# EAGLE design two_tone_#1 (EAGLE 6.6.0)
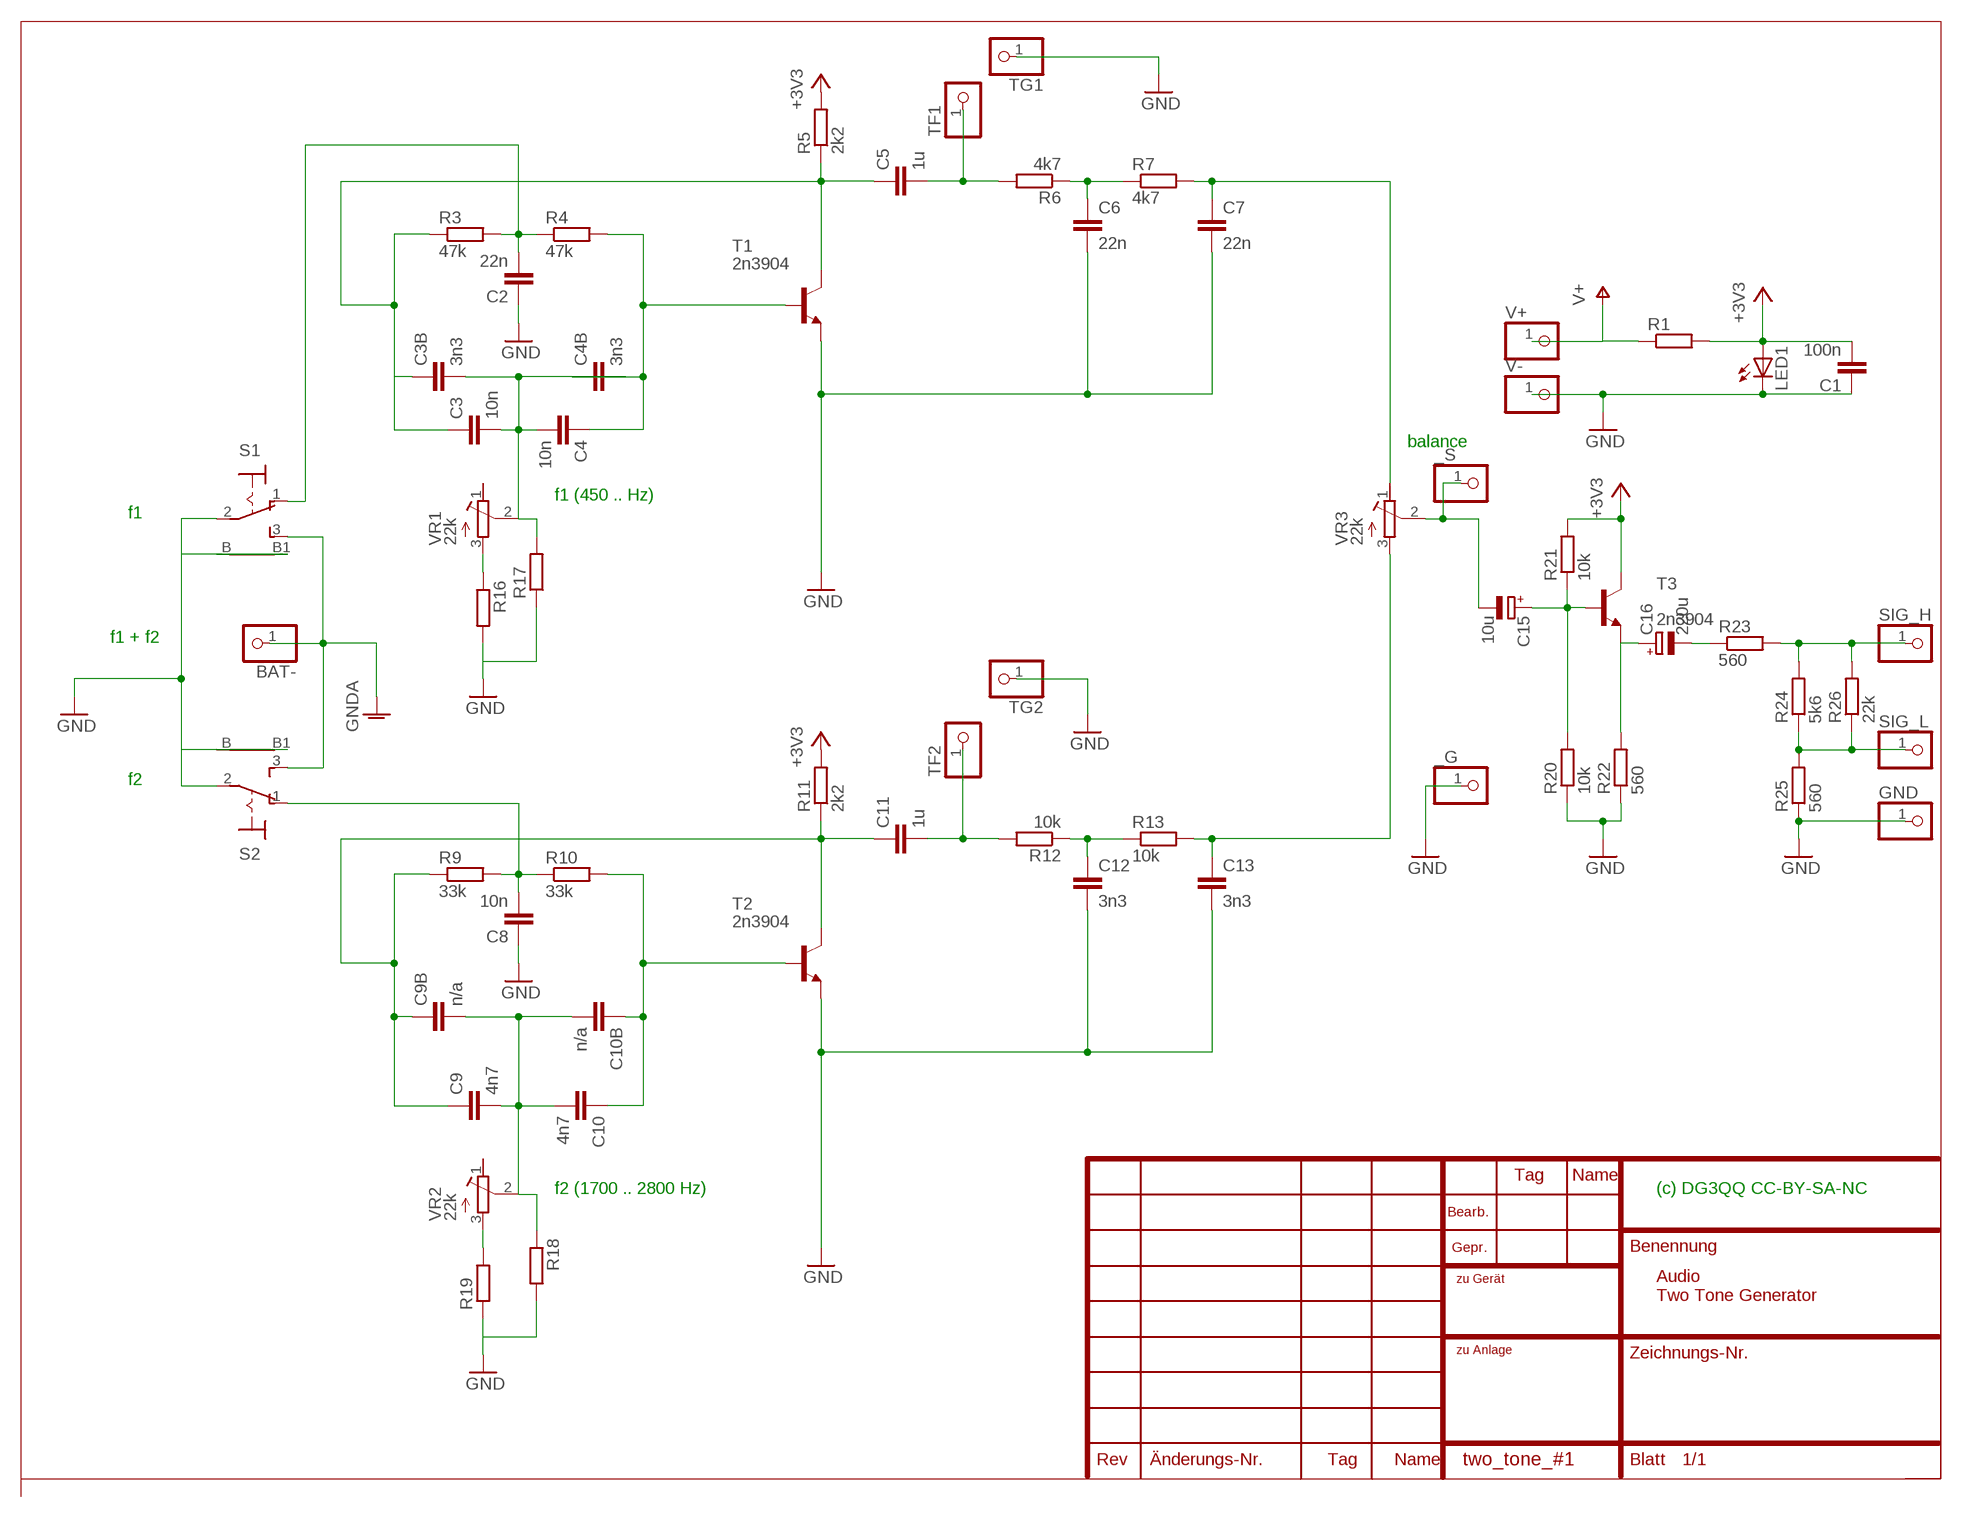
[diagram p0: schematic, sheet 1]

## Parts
_G  PINHD-1X1  [1X01]
_S  PINHD-1X1  [1X01]
BAT-  PINHD-1X1  [1X01]
C1  100n  C-EU025_050-025X075  [C025_050-025X075]
C2  22n  C-EU025_050-025X075  [C025_050-025X075]
C3  10n  C-EU025_050-025X075  [C025_050-025X075]
C3B  3n3  C-EU025_050-025X075  [C025_050-025X075]
C4  10n  C-EU025_050-025X075  [C025_050-025X075]
C4B  3n3  C-EU025_050-025X075  [C025_050-025X075]
C5  1u  C-EU025_050-025X075  [C025_050-025X075]
C6  22n  C-EU025_050-025X075  [C025_050-025X075]
C7  22n  C-EU025_050-025X075  [C025_050-025X075]
C8  10n  C-EU025_050-025X075  [C025_050-025X075]
C9  4n7  C-EU025_050-025X075  [C025_050-025X075]
C9B  n/a  C-EU025_050-025X075  [C025_050-025X075]
C10  4n7  C-EU025_050-025X075  [C025_050-025X075]
C10B  n/a  C-EU025_050-025X075  [C025_050-025X075]
C11  1u  C-EU025_050-025X075  [C025_050-025X075]
C12  3n3  C-EU025_050-025X075  [C025_050-025X075]
C13  3n3  C-EU025_050-025X075  [C025_050-025X075]
C15  10u  CPOL-EUE2.5-5  [E2,5-5]
C16  220u  CPOL-EUE5-10.5  [E5-10,5]
GND  PINHD-1X1  [1X01]
LED1  LED3MM  [LED3MM]
R1  R-EU_0207/2V  [0207/2V]
R3  47k  R-EU_0207/10  [0207/10]
R4  47k  R-EU_0207/2V  [0207/2V]
R5  2k2  R-EU_0207/2V  [0207/2V]
R6  4k7  R-EU_0207/2V  [0207/2V]
R7  4k7  R-EU_0207/2V  [0207/2V]
R9  33k  R-EU_0207/10  [0207/10]
R10  33k  R-EU_0207/2V  [0207/2V]
R11  2k2  R-EU_0207/2V  [0207/2V]
R12  10k  R-EU_0207/2V  [0207/2V]
R13  10k  R-EU_0207/2V  [0207/2V]
R16  R-EU_0207/2V  [0207/2V]
R17  R-EU_0207/2V  [0207/2V]
R18  R-EU_0207/2V  [0207/2V]
R19  R-EU_0207/2V  [0207/2V]
R20  10k  R-EU_0207/2V  [0207/2V]
R21  10k  R-EU_0207/2V  [0207/2V]
R22  560  R-EU_0207/2V  [0207/2V]
R23  560  R-EU_0207/2V  [0207/2V]
R24  5k6  R-EU_0207/2V  [0207/2V]
R25  560  R-EU_0207/2V  [0207/2V]
R26  22k  R-EU_0207/2V  [0207/2V]
S1  9070-1W  [9070-1W]
S2  9070-1W  [9070-1W]
SIG_H  PINHD-1X1  [1X01]
SIG_L  PINHD-1X1  [1X01]
T1  2n3904  2N3904-NPN-TO92-EBC  [TO92-EBC]
T2  2n3904  2N3904-NPN-TO92-EBC  [TO92-EBC]
T3  2n3904  2N3904-NPN-TO92-EBC  [TO92-EBC]
TF1  PINHD-1X1  [1X01]
TF2  PINHD-1X1  [1X01]
TG1  PINHD-1X1  [1X01]
TG2  PINHD-1X1  [1X01]
V+  PINHD-1X1  [1X01]
V-  PINHD-1X1  [1X01]
VR1  22k  R-TRIMM_414S6  [SPINDLE_414S6]
VR2  22k  R-TRIMM_414S6  [SPINDLE_414S6]
VR3  22k  R-TRIMM_414S6  [SPINDLE_414S6]

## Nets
+3V3: C1.2 LED1.A R1.2 R5.2 R11.2 R21.2 T3.C
BAT-: BAT-.1 S1.3(S) S2.3(S) ; supply symbol labelled GNDA
GND: _G.1 C1.1 C2.1 C6.2 C7.2 C8.1 C12.2 C13.2 GND.1 LED1.K(C) R16.2 R17.1 R18.2 R19.1 R20.1 R22.1 R25.1 S1.2(P) S1.B S1.B1 S2.2(P) S2.B S2.B1 T1.E T2.E TG1.1 TG2.1 V-.1
N$1: C5.2 R6.2 TF1.1
N$2: C6.1 R6.1 R7.1
N$3: C2.2 R3.2 R4.1 S1.1(O)
N$4: C4.1 C4B.1 R4.2 T1.B
N$5: C3.1 C3B.1 C5.1 R3.1 R5.1 T1.C
N$6: C3.2 C3B.2 C4.2 C4B.2 R17.2 VR1.2(S)
N$7: C7.1 R7.2 VR3.1(A)
N$8: C8.2 R9.2 R10.1 S2.1(O)
N$9: C10.1 C10B.1 R10.2 T2.B
N$10: C9.1 C9B.1 C11.1 R9.1 R11.1 T2.C
N$11: C9.2 C9B.2 C10.2 C10B.2 R18.1 VR2.2(S)
N$12: C11.2 R12.2 TF2.1
N$13: C12.1 R12.1 R13.1
N$14: C13.1 R13.2 VR3.3(E)
N$15: R19.2 VR2.3(E)
N$16: C15.+ R20.2 R21.1 T3.B
N$17: _S.1 C15.- VR3.2(S)
N$19: R16.1 VR1.3(E)
N$20: C16.+ R22.2 T3.E
N$23: C16.- R23.1
N$24: R23.2 R24.2 R26.2 SIG_H.1
N$25: R24.1 R25.2 R26.1 SIG_L.1
V+: R1.1 V+.1
Unconnected: VR1.1(A) VR2.1(A)

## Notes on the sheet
- balance
- f1 (450 .. Hz)
- f1
- f1 + f2
- f2
- f2 (1700 .. 2800 Hz) | (c) DG3QQ CC-BY-SA-NC
- Audio 
  Two Tone Generator

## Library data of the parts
_G _S BAT- GND SIG_H SIG_L TF1 TF2 TG1 TG2 V+ V- = pinhead:PINHD-1X1: PIN HEADER
C1-C3 C3B C4 C4B C5-C9 C9B C10 C10B C11-C13 = resistor:C-EU: CAPACITOR, European symbol
C15 C16 = resistor:CPOL-EU: POLARIZED CAPACITOR, European symbol
LED1 = led:LED: LED
R1 R3-R7 R9-R13 R16-R26 = resistor:R-EU_: RESISTOR, European symbol
S1 S2 = switch:9070-1W: TOGGLE SWITCH Marquardt
T1-T3 = transistor-neu-to92:*-NPN-: NPN Transistror
VR1-VR3 = dg3qq_:R-TRIMM_414S6

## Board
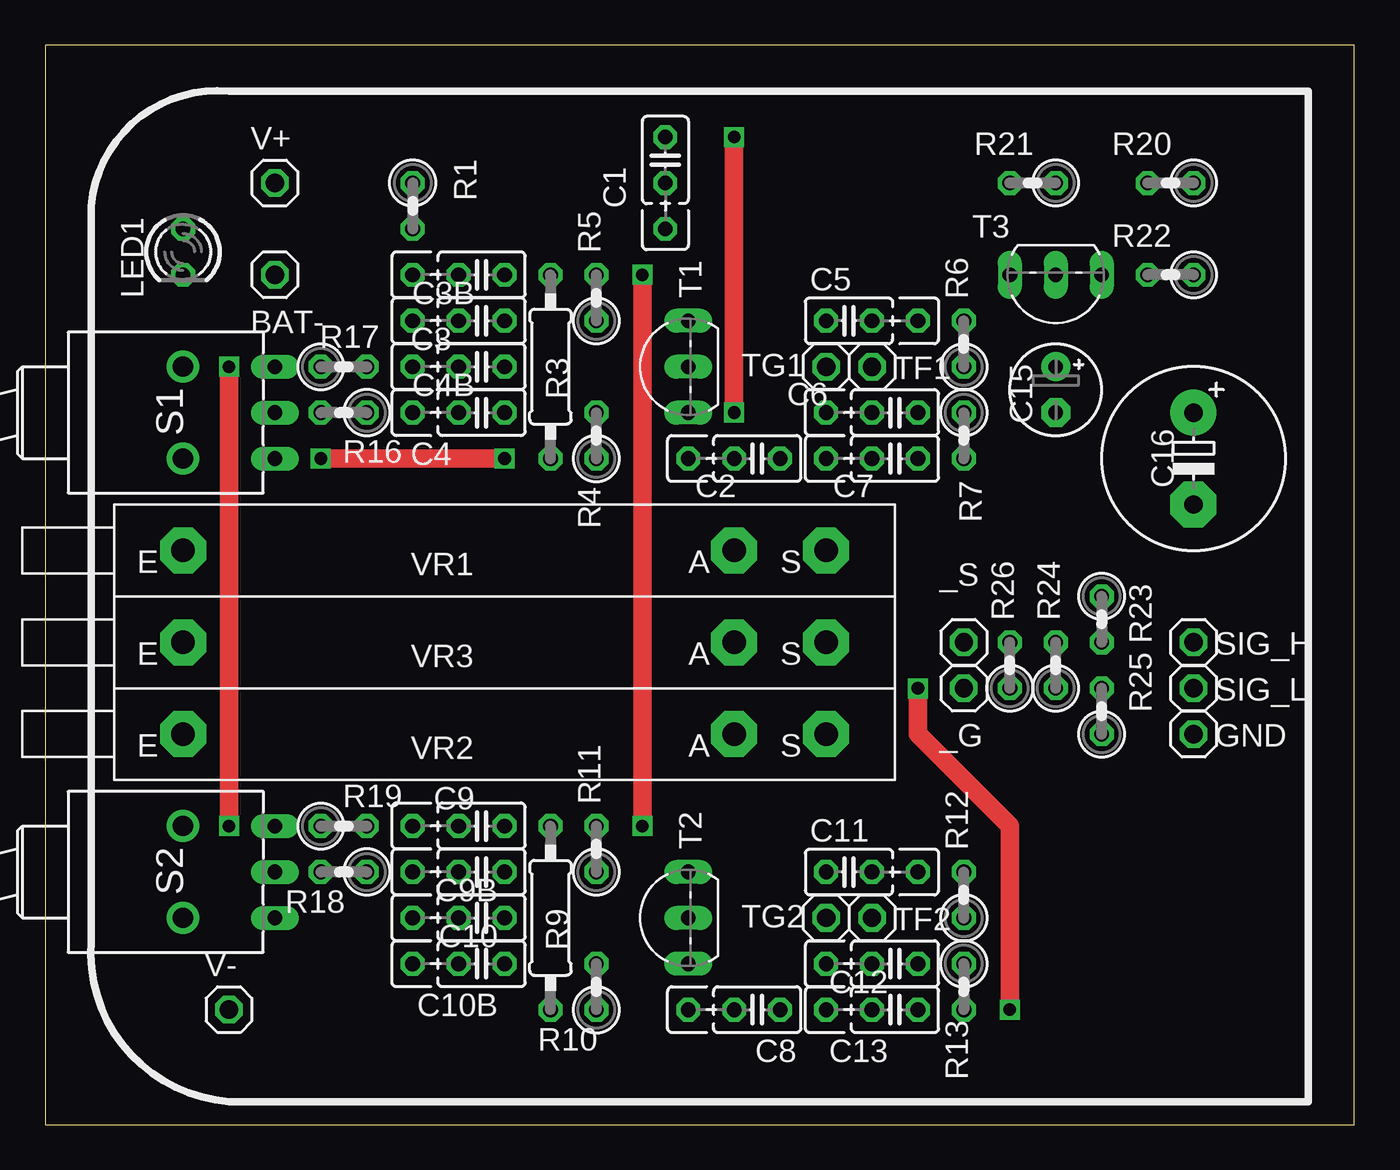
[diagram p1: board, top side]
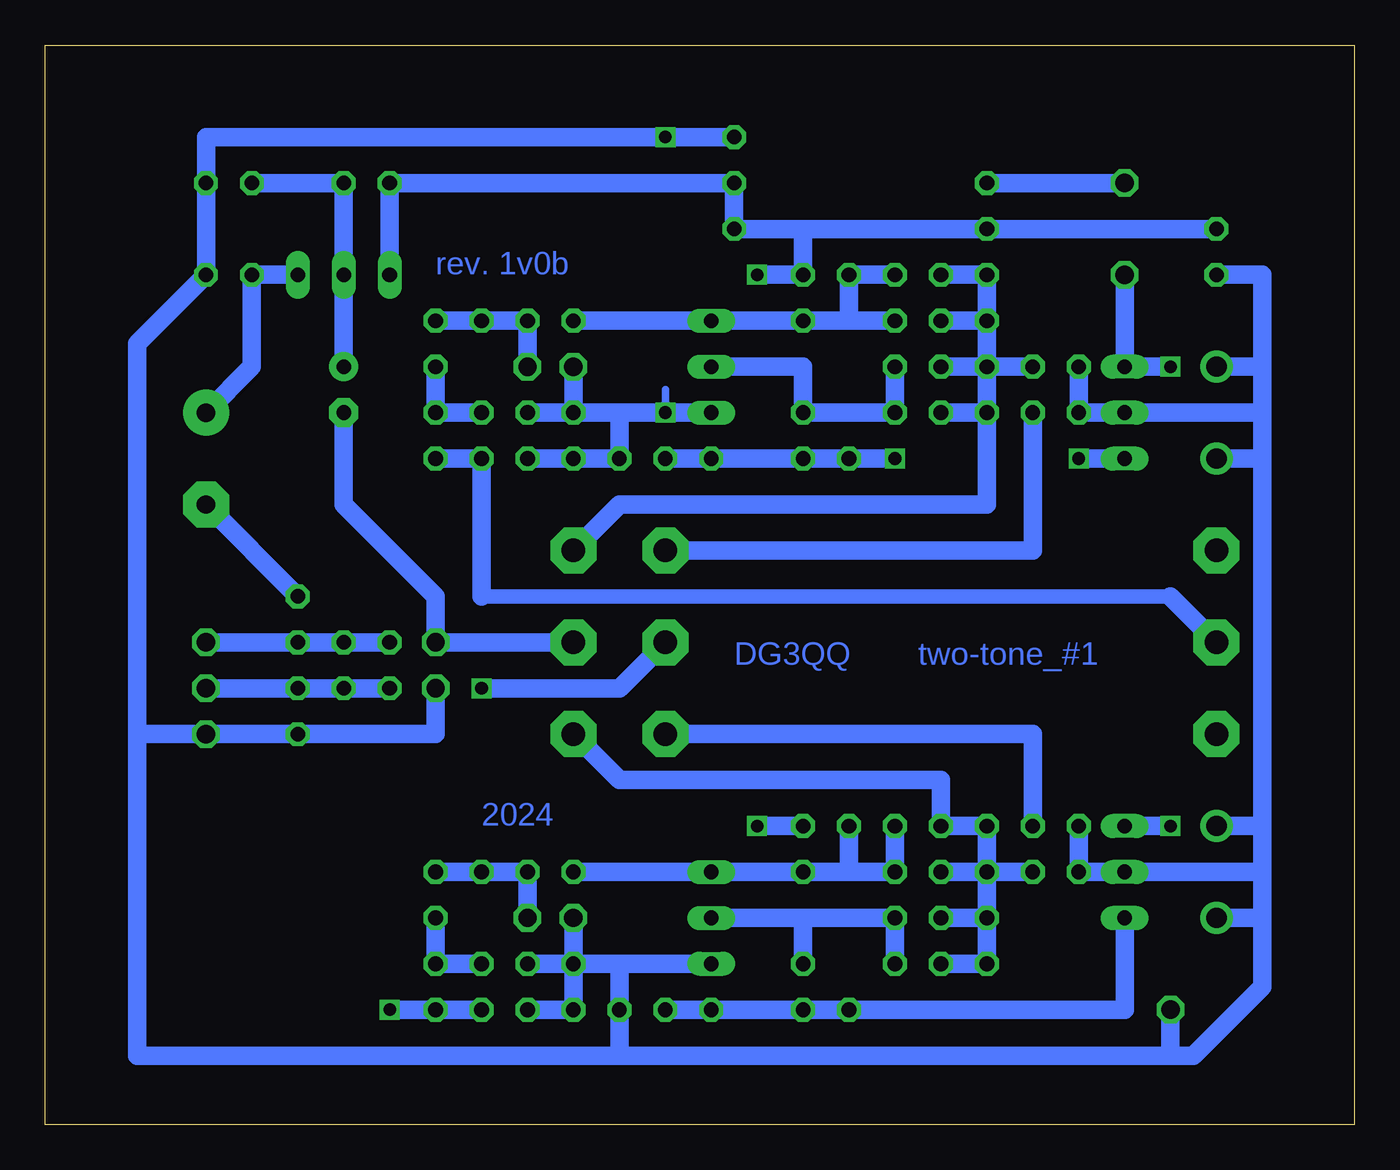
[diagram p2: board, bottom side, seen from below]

Size 72.39 x 59.69 mm. Coordinates in mm from the lower left corner, seen from the top.
Outline: 0,0 72.39,0 72.39,59.69 0,59.69 0,0
Copper layers (1*16): Top 0.035mm / dielectric 1.5mm / Bottom 0.035mm
Design rules "default": minimum track width 10mil, minimum drill 24mil, track to track 8mil, track to pad 8mil, pad to pad 8mil, via to via 8mil, smd to smd 8mil, copper to edge 40mil, drill to drill 8mil, minimum pad ring 10mil, minimum via ring 8mil, stop-mask expansion 4mil, vias tented up to drill 0mil, thermal gap 10mil

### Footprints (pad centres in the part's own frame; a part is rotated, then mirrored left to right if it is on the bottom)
1X01 = drill 1.016 octagon: 1 0,0
C025_050-025X075 = drill 0.813 octagon: 1 -1.27,0; 2 1.27,0; 3 3.81,0
E2,5-5 = drill 0.813 pad 1.6: + -1.27,0 | drill 0.813 pad 1.6 octagon: - 1.27,0
E5-10,5 = drill 1.016 pad 2.54: + -2.54,0 | drill 1.016 pad 2.54 octagon: - 2.54,0
LED3MM = drill 0.813 octagon: A -1.27,0; K 1.27,0
0207/2V = drill 0.813 octagon: 1 -1.27,0; 2 1.27,0
0207/10 = drill 0.813 octagon: 1 -5.08,0; 2 5.08,0
9070-1W = drill 0.813 long: 1 5.08,-2.54; 2 5.08,0; 3 5.08,2.54 | drill 1.118 pad 1.778: B 0,-2.54; B1 0,2.54
TO92-EBC = drill 0.813 long: B 0,-1.27; C 2.54,-1.27; E -2.54,-1.27
SPINDLE_414S6 = drill 1.3 pad 2.54 octagon: 1 -2.54,0; 2 33.02,0; 3 27.94,0

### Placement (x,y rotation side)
_G  50.8,24.13 0 top
_S  50.8,26.67 0 top
BAT-  12.7,46.99 0 top
C1  34.29,53.34 270 top
C2  39.37,36.83 180 top
C3  24.13,44.45 180 top
C3B  24.13,46.99 180 top
C4  24.13,39.37 180 top
C4B  24.13,41.91 180 top
C5  44.45,44.45 0 top
C6  46.99,39.37 180 top
C7  46.99,36.83 180 top
C8  39.37,6.35 180 top
C9  24.13,16.51 180 top
C9B  24.13,13.97 180 top
C10  24.13,11.43 180 top
C10B  24.13,8.89 180 top
C11  44.45,13.97 0 top
C12  46.99,8.89 180 top
C13  46.99,6.35 180 top
C15  55.88,40.64 270 top
C16  63.5,36.83 270 top
GND  63.5,21.59 0 top
LED1  7.62,48.26 270 top
R1  20.32,50.8 270 top
R3  27.94,41.91 270 top
R4  30.48,38.1 90 top
R5  30.48,45.72 90 top
R6  50.8,43.18 90 top
R7  50.8,38.1 270 top
R9  27.94,11.43 270 top
R10  30.48,7.62 90 top
R11  30.48,15.24 90 top
R12  50.8,12.7 90 top
R13  50.8,7.62 270 top
R16  16.51,39.37 180 top
R17  16.51,41.91 0 top
R18  16.51,13.97 180 top
R19  16.51,16.51 0 top
R20  62.23,52.07 180 top
R21  54.61,52.07 180 top
R22  62.23,46.99 180 top
R23  58.42,27.94 270 top
R24  55.88,25.4 90 top
R25  58.42,22.86 90 top
R26  53.34,25.4 90 top
S1  7.62,39.37 0 top
S2  7.62,13.97 0 top
SIG_H  63.5,26.67 0 top
SIG_L  63.5,24.13 0 top
T1  34.29,41.91 90 top
T2  34.29,11.43 90 top
T3  55.88,45.72 180 top
TF1  45.72,41.91 0 top
TF2  45.72,11.43 0 top
TG1  43.18,41.91 0 top
TG2  43.18,11.43 0 top
V+  12.7,52.07 0 top
V-  10.16,6.35 0 top
VR1  10.16,31.75 0 top
VR2  10.16,21.59 0 top
VR3  10.16,26.67 0 top

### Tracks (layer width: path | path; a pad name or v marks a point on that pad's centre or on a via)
+3V3  (via drill 0.7)
  Top 1.016: v33.02,46.99 v33.02,16.51
  Bottom 1.016: LED1.A R1.2 30.48,49.53 | T3.C R21.2 C1.2 34.29,49.53 30.48,49.53 | 30.48,49.53 R5.2 v33.02,46.99 | v33.02,16.51 R11.2
BAT-  (via drill 0.7)
  Top 1.016: v10.16,41.91 v10.16,16.51
  Bottom 1.016: BAT-.1 S1.3 v10.16,41.91 | v10.16,16.51 S2.3
GND  (via drill 0.7)
  Top 1.016: v38.1,54.61 v38.1,39.37
  Bottom 0.406: v38.1,39.37 38.1,40.64 | 6.35,41.91 S1.B1
  Bottom 1.016: T1.E v38.1,39.37 40.64,39.37 | C6.2 43.18,39.37 | 40.64,3.81 67.31,3.81 67.31,21.59 | 40.64,3.81 C8.1 40.64,8.89 | 10.16,3.81 8.89,3.81 5.08,7.62 5.08,11.43 | 10.16,3.81 40.64,3.81 | 5.08,36.83 5.08,16.51 | S1.B 5.08,36.83 | 5.08,36.83 5.08,39.37 | 5.08,39.37 5.08,41.91 | 5.08,41.91 S1.B1 | 40.64,39.37 C2.1 C7.2 | C1.1 v38.1,54.61 63.5,54.61 R20.1 R22.1 67.31,43.18 67.31,21.59 | 5.08,41.91 5.08,46.99 LED1.K | 5.08,13.97 5.08,11.43 | 5.08,11.43 S2.B | 5.08,39.37 S1.2 R16.2 R17.1 | S2.B1 5.08,16.51 | 5.08,16.51 5.08,13.97 | 5.08,13.97 R18.2 | R18.2 R19.1 | R18.2 S2.2 | 67.31,21.59 GND.1 R25.1 50.8,21.59 _G.1 | 40.64,39.37 43.18,39.37 | 43.18,39.37 TG1.1 | V-.1 10.16,3.81 | 43.18,8.89 43.18,6.35 C13.2 | 40.64,8.89 43.18,8.89 | 43.18,8.89 TG2.1 | T2.E 40.64,8.89 | 43.18,8.89 C12.2
N$1
  Bottom 1.016: R6.2 C5.2 TF1.1
N$2
  Bottom 1.016: R6.1 R7.1 C6.1
N$3  (via drill 0.7)
  Top 1.016: v25.4,36.83 v15.24,36.83
  Bottom 1.016: C2.2 R4.1 R3.2 v25.4,36.83 | S1.1 v15.24,36.83
N$4
  Bottom 1.016: T1.B 30.48,41.91 R4.2 C4.1 C4B.1
N$5
  Bottom 1.016: C3.1 27.94,44.45 | 27.94,44.45 R5.1 T1.C C5.1 | C3B.1 R3.1 27.94,44.45
N$6
  Bottom 1.016: C4B.2 20.32,41.91 | 20.32,41.91 20.32,39.37 | C4.2 20.32,39.37 | 20.32,39.37 20.32,34.29 40.64,34.29 VR1.2 | R17.2 20.32,41.91 | 20.32,44.45 20.32,41.91 | C3B.2 20.32,46.99 20.32,44.45 | 20.32,44.45 C3.2
N$7
  Bottom 0.813: 48.26,29.21 10.16,29.21
  Bottom 1.016: 48.26,29.21 C7.1 R7.2 | 10.16,29.21 VR3.1
N$8
  Bottom 1.016: C8.2 R10.1 R9.2 12.7,6.35 S2.1
N$9
  Bottom 1.016: T2.B 30.48,11.43 | R10.2 30.48,11.43 | 30.48,11.43 C10.1 C10B.1
N$10
  Bottom 1.016: 27.94,13.97 C9B.1 C9.1 | 27.94,13.97 R11.1 T2.C C11.1 | 27.94,13.97 R9.1
N$11
  Bottom 1.016: 20.32,13.97 20.32,16.51 C9.2 22.86,19.05 40.64,19.05 VR2.2 | 20.32,11.43 20.32,13.97 | 20.32,13.97 C9B.2 R18.1 | C10.2 20.32,11.43 | 20.32,11.43 20.32,8.89 C10B.2
N$12
  Bottom 1.016: TF2.1 C11.2 R12.2
N$13
  Bottom 1.016: R12.1 R13.1 C12.1
N$14  (via drill 0.7)
  Top 1.016: v53.34,6.35 53.34,16.51 48.26,21.59 v48.26,24.13
  Bottom 1.016: R13.2 C13.1 v53.34,6.35 | v48.26,24.13 40.64,24.13 VR3.3
N$15
  Bottom 1.016: VR2.3 17.78,21.59 R19.2
N$16
  Bottom 1.016: R20.2 R21.1 T3.B C15.+
N$17
  Bottom 1.016: VR3.2 _S.1 50.8,29.21 55.88,34.29 C15.-
N$19
  Bottom 1.016: VR1.3 17.78,31.75 R16.1
N$20
  Bottom 1.016: T3.E R22.2 60.96,41.91 C16.+
N$23
  Bottom 1.016: R23.1 C16.-
N$24
  Bottom 1.016: SIG_H.1 R23.2 R24.2 R26.2
N$25
  Bottom 1.016: SIG_L.1 R25.2 R24.1 R26.1
V+
  Bottom 1.016: V+.1 R1.1

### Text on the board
Bottom: rev. 1v0b | two-tone_#1 | DG3QQ | 2024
